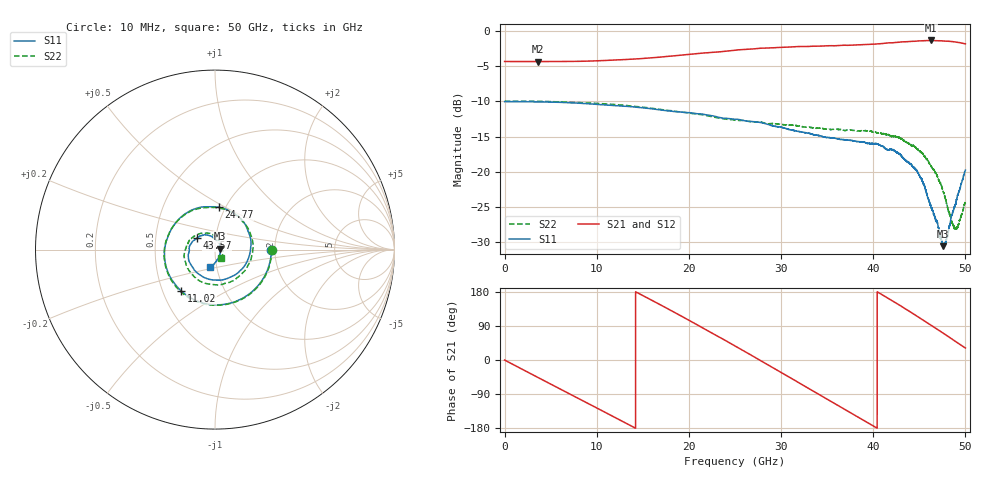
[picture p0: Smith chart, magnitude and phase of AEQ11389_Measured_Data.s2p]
!Keysight Technologies,N5227B,US61251182,A.15.40.08
!Date: Friday, November 24, 2023 09:04:31
!Correction: S11(C  2-Port  )
!S21(C  2-Port  )
!S12(C  2-Port  )
!S22(C  2-Port  )
!S2P File: Measurements: S11, S21, S12, S22:
# Hz S  dB  R 50
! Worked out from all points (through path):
!   12801 points, 10 MHz to 50 GHz, reference 50 ohm
!   highest |S21| = -1.39 dB at 46.3 GHz (marker M1); lowest = -4.4 dB at 3.587 GHz (marker M2)
!   group delay of S21, straight-line fit = 37.9 ps
!   lowest |S11| = -30.5 dB at 47.55 GHz (marker M3), VSWR 1.06, Z = 53 + j0.648 ohm
!   |S11| at or under -10 dB: start of sweep to end of sweep
!   |S22| runs from -28.1 to -10.0 dB; largest |S21 - S12| = 1.6
!   S11 on the Smith chart (normalised r, x): 10 MHz: 1.92, -0.00; 11.02 GHz: 0.62, -0.31; 24.77 GHz: 0.93, +0.46; 43.57 GHz: 0.81, +0.10; 50 GHz: 0.93, -0.19
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1e7  -10.06 -0.0  -4.37 -0.1  -4.38 -0.1  -10.00 -0.1
3.587409e9  -10.10 -43.6  -4.39 -45.6  -4.38 -34.6  -10.01 -42.9
6.012705e9  -10.16 -72.5  -4.37 -76.3  -4.37 -57.9  -10.10 -71.4
8.34427e9  -10.29 -99.6  -4.34 -105.7  -4.34 -80.1  -10.20 -98.1
1.101561e10  -10.53 -129.4  -4.22 -139.3  -4.22 -105.6  -10.37 -127.7
1.389394e10  -10.78 -160.3  -4.04 -175.9  -4.04 -133.4  -10.70 -158.3
1.667464e10  -11.19 170.8  -3.78 148.6  -3.78 -160.3  -11.10 172.6
2.093941e10  -11.77 126.9  -3.24 92.3  -3.24 156.4  -11.84 128.2
2.477458e10  -12.53 84.9  -2.81 40.4  -2.82 116.2  -12.64 87.9
2.5005e10  -12.56 82.4  -2.78 37.2  -2.78 113.7  -12.68 85.4
2.706709e10  -12.90 57.4  -2.58 8.5  -2.58 91.3  -12.92 62.8
2.894952e10  -13.43 31.5  -2.44 -18.0  -2.44 70.6  -13.17 39.9
3.141387e10  -14.14 -4.2  -2.29 -52.6  -2.29 43.5  -13.41 7.2
3.333927e10  -14.66 -35.9  -2.22 -79.8  -2.22 22.2  -13.74 -20.3
3.553805e10  -15.17 -73.3  -2.14 -110.9  -2.14 -2.2  -14.00 -52.4
3.813909e10  -15.70 -118.8  -2.03 -147.6  -2.03 -30.9  -14.20 -92.8
4.166964e10  -16.89 -178.9  -1.74 162.0  -1.74 -70.5  -14.77 -150.7
4.356769e10  -18.42 148.5  -1.57 133.8  -1.58 -92.9  -15.78 177.0
4.630152e10  -25.11 87.0  -1.39 91.4  -1.40 -126.9  -19.24 123.3
4.755127e10  -30.53 11.8  -1.46 71.4  -1.47 -143.1  -22.65 89.2
4.887913e10  -24.71 -77.5  -1.60 49.7  -1.61 -160.7  -27.92 19.5
5e10  -19.76 -104.4  -1.87 31.5  -1.87 -175.4  -24.43 -54.3
